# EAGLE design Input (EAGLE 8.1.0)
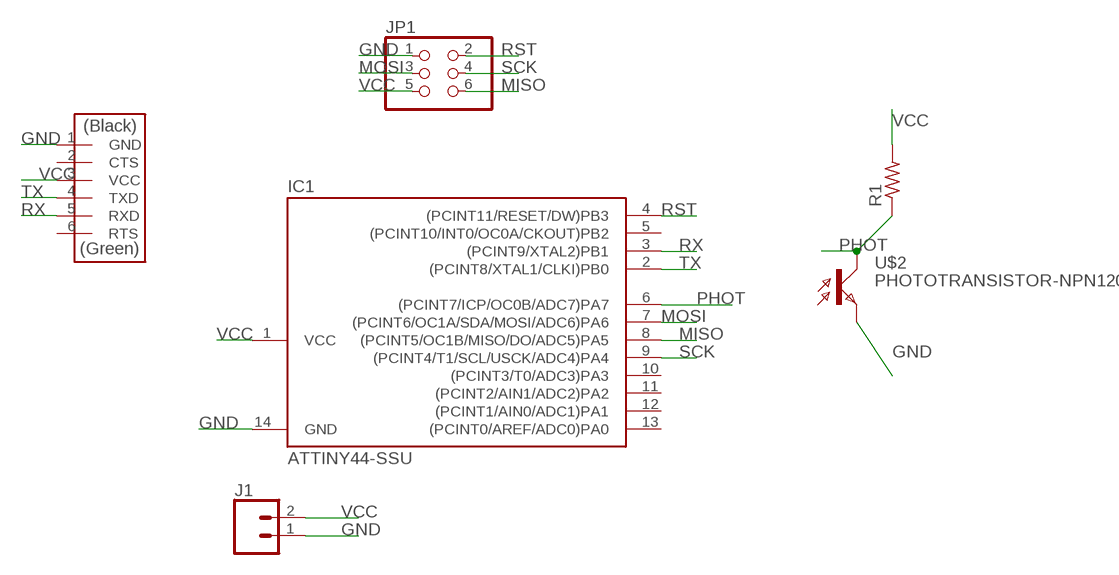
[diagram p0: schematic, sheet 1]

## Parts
IC1  ATTINY44-SSU  [SOIC14]
J1  CONN_02PTH3  [1X02_LONGPADS]
JP1  PINHD-2X3-SMD  [2X03SMD]
R1  RES-US1206FAB  [R1206FAB]
U$2  PHOTOTRANSISTOR-NPN1206  [OP1206]
U$4  FTDI-SMD-HEADER  [1X06SMD]

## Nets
GND: IC1.14(GND) J1.1 JP1.1 U$2.EMITTER(E) U$4.1(GND)
MISO: IC1.8((PCINT5/OC1B/MISO/DO/ADC5)PA5) JP1.6
MOSI: IC1.7((PCINT6/OC1A/SDA/MOSI/ADC6)PA6) JP1.3
PHOT: IC1.6((PCINT7/ICP/OC0B/ADC7)PA7) R1.1 U$2.COLLECTOR(C)
RST: IC1.4((PCINT11/RESET/DW)PB3) JP1.2
RX: IC1.3((PCINT9/XTAL2)PB1) U$4.5(RXD)
SCK: IC1.9((PCINT4/T1/SCL/USCK/ADC4)PA4) JP1.4
TX: IC1.2((PCINT8/XTAL1/CLKI)PB0) U$4.4(TXD)
VCC: IC1.1(VCC) J1.2 JP1.5 R1.2 U$4.3(VCC)
Unconnected: IC1.5((PCINT10/INT0/OC0A/CKOUT)PB2) IC1.10((PCINT3/T0/ADC3)PA3) IC1.11((PCINT2/AIN1/ADC2)PA2) IC1.12((PCINT1/AIN0/ADC1)PA1) IC1.13((PCINT0/AREF/ADC0)PA0) U$4.2(CTS) U$4.6(RTS)

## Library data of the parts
IC1 = fab:ATTINY44
J1 = SparkFun-Connectors:CONN_02: Multi connection point. Often used as Generic Header-pin footprint for 0.1 inch spaced/style header connections
JP1 = fab:PINHD-2X3-SMD: PIN HEADER
R1 = fab:RES-US: Resistor (US Symbol)
U$2 = fab:PHOTOTRANSISTOR-NPN
U$4 = fab:FTDI-SMD-HEADER

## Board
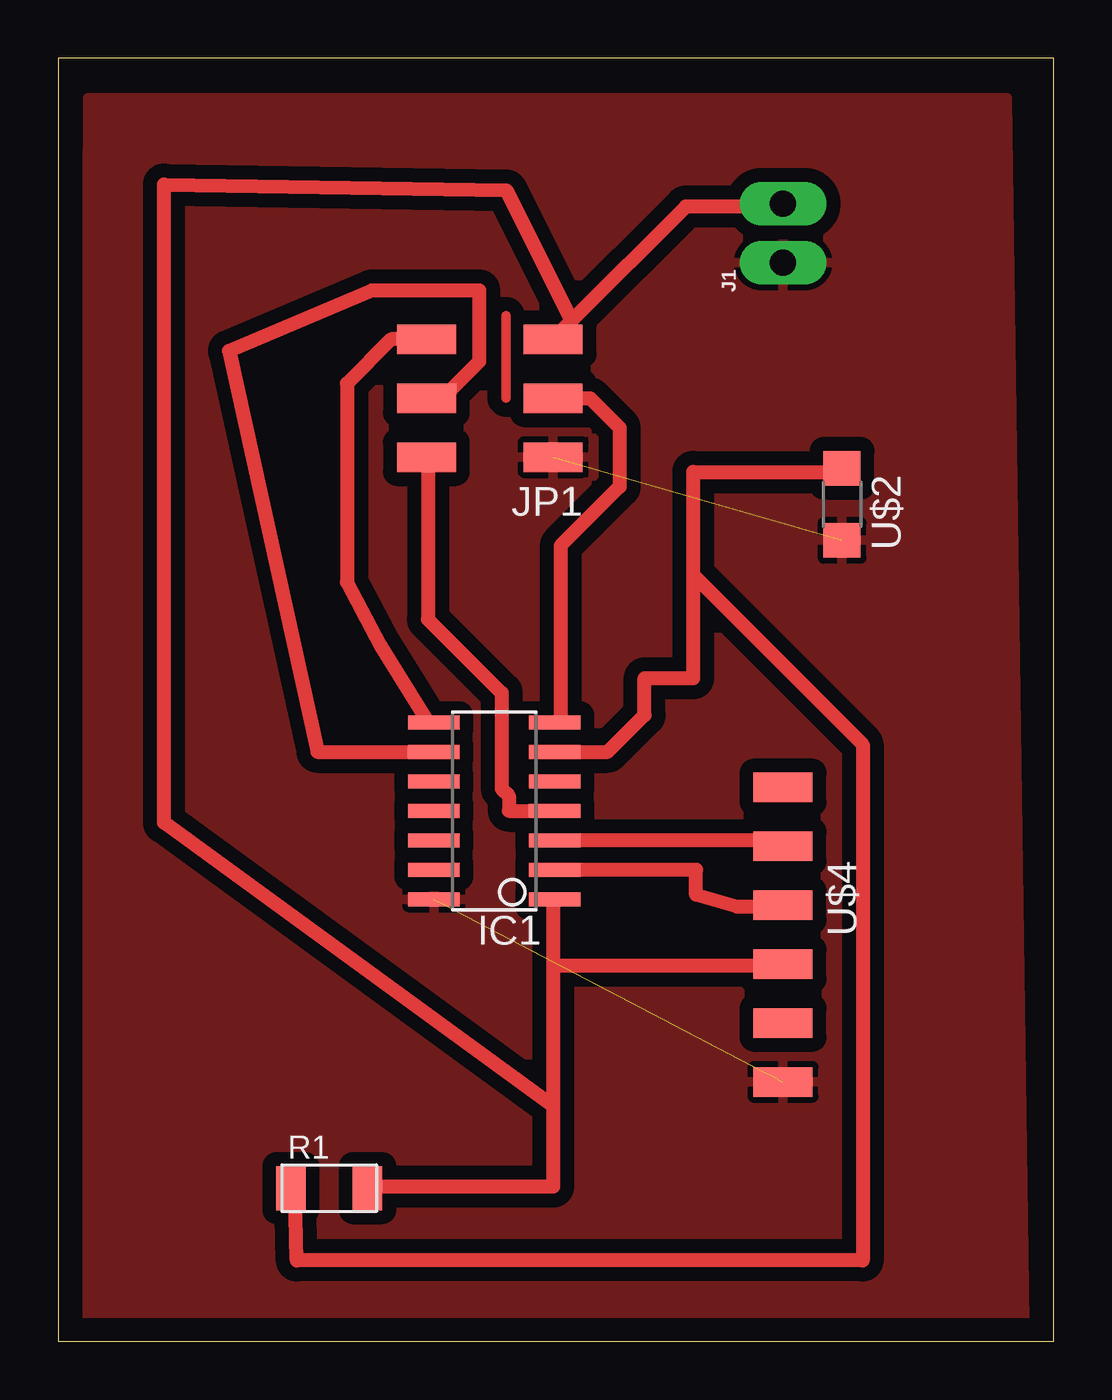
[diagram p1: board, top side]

Size 42.91 x 55.3 mm. Coordinates in mm from the lower left corner, seen from the top.
Outline: 0,0 42.91,0 42.91,55.3 0,55.3 0,0
Copper layers (1*16): Top 0.4mm / dielectric 0.4mm / Bottom 0.4mm
Design rules "default *": minimum track width 0.6mm, minimum drill 24mil, track to track 0.6mm, track to pad 0.6mm, pad to pad 0.6mm, via to via 8mil, smd to smd 8mil, copper to edge 40mil, drill to drill 8mil, minimum pad ring 10mil, minimum via ring 8mil, stop-mask expansion 4mil, vias tented up to drill 0mil, thermal gap 10mil

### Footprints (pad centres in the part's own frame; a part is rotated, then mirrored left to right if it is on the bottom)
SOIC14 = smd 0.61 x 2.21: 1 -3.81,-2.603; 2 -2.54,-2.603; 3 -1.27,-2.603; 4 0,-2.603; 5 1.27,-2.603; 6 2.54,-2.603; 7 3.81,-2.603; 8 3.81,2.603; 9 2.54,2.603; 10 1.27,2.603; 11 0,2.603; 12 -1.27,2.603; 13 -2.54,2.603; 14 -3.81,2.603
1X02_LONGPADS = drill 1.118 pad 1.88 long: 1 0,0; 2 2.54,0
2X03SMD = smd 2.54 x 1.27: 1 -2.54,2.54; 2 2.92,2.54; 3 -2.54,0; 4 2.92,0; 5 -2.54,-2.54; 6 2.92,-2.54
R1206FAB = smd 1.27 x 1.905: 1 -1.651,0; 2 1.651,0
OP1206 = smd 1.5 x 1.6: COLLECTOR -1.55,0; EMITTER 1.55,0
1X06SMD = smd 2.54 x 1.27: 1 0,6.35; 2 0,3.81; 3 0,1.27; 4 0,-1.27; 5 0,-3.81; 6 0,-6.35

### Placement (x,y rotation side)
IC1  18.8,22.86 90 top
J1  31.24,46.48 90 top
JP1  18.8,40.64 180 top
R1  11.68,6.6 0 top
U$2  33.78,36.07 270 top
U$4  31.24,17.53 180 top

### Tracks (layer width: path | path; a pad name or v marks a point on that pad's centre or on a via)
GND  (2 unrouted)
  pour Top: 1.27,53.59 40.89,53.59 41.66,0.76 1.02,0.51
MISO
  Top 0.6: JP1.6 14.35,43.18 12.45,41.27 12.45,32.7 13.91,29.97 15.94,26.67 IC1.8
MOSI
  Top 0.6: JP1.3 22.92,40.64 24.19,39.37 24.19,36.83 21.65,34.29 21.65,26.67 IC1.7
N$1
  Top 0.406: 19.3,44.2 19.3,40.64
PHOT
  Top 0.6: IC1.6 23.69,25.4 25.27,26.99 25.27,28.58 27.37,28.58 27.37,33.02 | 27.37,33.02 27.37,37.46 33.72,37.46 U$2.COLLECTOR | 27.37,33.02 34.67,25.72 34.67,3.49 10.29,3.49 10.22,6.35 R1.1
RST
  Top 0.6: 15.62,38.1 JP1.2 15.94,38.1 15.94,31.12 19.11,27.94 19.11,23.81 19.43,23.49 19.43,22.86 IC1.4
RX
  Top 0.6: IC1.3 31.18,21.59 U$4.5
SCK
  Top 0.6: IC1.9 11.18,25.4 7.37,42.67 13.53,45.28 18.16,45.28 18.16,42.23 16.57,40.64 JP1.4
TX
  Top 0.6: IC1.2 27.49,20.32 27.49,19.24 29.27,18.73 31.18,18.73 U$4.4
VCC
  Top 0.6: 22.13,43.97 27.05,48.89 31.18,48.89 J1.2 | 22.13,43.97 JP1.5 | 21.34,16.19 21.34,19.05 IC1.1 | 21.34,16.19 21.34,10.16 | 21.34,10.16 21.34,6.67 13.4,6.67 R1.2 | 21.34,16.19 31.18,16.19 U$4.3 | 22.13,43.97 19.3,49.59 4.57,49.85 4.57,22.35 21.34,10.16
